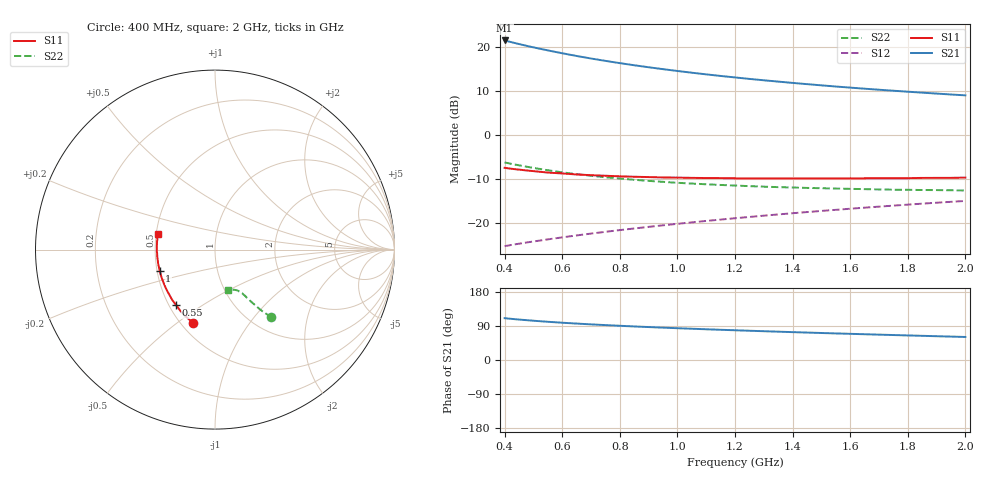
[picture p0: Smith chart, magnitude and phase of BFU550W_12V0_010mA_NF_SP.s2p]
! Filename:  P:\Prog\Test\Noise\ATS_data\Testdata_Net\06 Compressed Noise after Statistics\BFU550W_APM2013_11_D05_12p0V_010mA_NF_CM01_D.sf
! Date/Time: Tue 26/Mar/2013 16:25:26
! BFU550W_APM2013_11_D05_12p0V_1to35mA_NF_CM01_Bias6_R.sf
! Noise Parameter Data File
! BFU550W_APM2013_11_D05_12p0V_1to35mA_NF_CM01
! Date/time: Mon Mar 25 15:58:35 2013
! VAR V_out= 12.001000
! VAR I_out= 9.990000
! VAR V_in= 0.792300
! VAR I_in= 0.086905
! Device data file deembeded for feedlines and parallel
! Original file: \06 Compressed Noise after Statistics\BFU550W_APM2013_11_D05_12p0V_010mA_NF_CM01_R.sf
! Feed-files: PR019V01_070313_Feed1.s2p, PR019V01_070313_Feed2.s2p
! Parallel-file: PR019V01_070313_Par.s2p
# MHz S MA R 50
!  Freq-MHz  S11-mag  S11-arg  S21-mag  S21-arg  S12-mag  S12-arg  S22-mag  S22-arg
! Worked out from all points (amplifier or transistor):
!   37 points, 400 MHz to 2 GHz, reference 50 ohm
!   highest |S21| = 21.5 dB at 400 MHz (marker M1)
!   |S21| within 3 dB of that: start of sweep to 608.1 MHz
!   unconditionally stable (mu >= 1): 1.474 GHz to end of sweep
!   at 500 MHz: K = 0.72, MSG = 22.0 dB, |S12| = -24.1 dB
!   at 1.1 GHz: K = 0.96, MSG = 16.6 dB, |S12| = -19.4 dB
!   at 2 GHz: K = 1.01, MAG = 11.3 dB, |S12| = -14.9 dB
!   lowest NFmin = 0.73 dB at 420 MHz
!   S11 on the Smith chart (normalised r, x): 400 MHz: 0.57, -0.57; 550 MHz: 0.54, -0.39; 1 GHz: 0.52, -0.14; 2 GHz: 0.51, +0.10
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400  0.4265 -106.5  11.85 110.3  0.05524 58.0  0.4904 -50.1
420  0.4181 -109.3  11.4 108.8  0.05674 57.9  0.476 -50.7
440  0.4105 -112.1  10.99 107.4  0.0582 57.9  0.462 -51.3
460  0.4038 -114.7  10.6 106.1  0.05964 58.0  0.4491 -51.8
500  0.3914 -119.7  9.892 103.7  0.06244 58.2  0.4258 -52.7
550  0.377 -125.1  9.144 100.9  0.06595 58.6  0.4006 -53.6
600  0.3684 -130.2  8.482 98.4  0.06951 59.0  0.3792 -54.2
650  0.3589 -134.7  7.902 96.1  0.07309 59.4  0.3623 -54.9
700  0.3522 -139.0  7.397 94.0  0.07669 59.9  0.3469 -55.5
750  0.347 -142.8  6.952 92.1  0.08034 60.3  0.3337 -55.9
800  0.3417 -146.5  6.556 90.3  0.08401 60.7  0.3227 -56.5
850  0.338 -150.0  6.202 88.5  0.08766 61.1  0.3122 -56.8
950  0.3319 -155.9  5.601 85.4  0.09519 61.8  0.2959 -57.6
1000  0.3305 -158.7  5.343 83.9  0.09898 62.0  0.2887 -57.9
1100  0.3268 -163.8  4.891 81.1  0.1067 62.5  0.2778 -59.0
1200  0.3248 -168.4  4.513 78.5  0.1145 62.8  0.2687 -60.1
1250  0.3241 -170.8  4.343 77.2  0.1184 62.9  0.2645 -60.5
1350  0.3235 -174.6  4.047 74.7  0.1265 63.1  0.2578 -61.7
1500  0.3236 179.8  3.672 71.2  0.1386 63.0  0.2507 -63.7
1650  0.3248 174.6  3.364 68.0  0.1509 62.9  0.2447 -65.7
1750  0.3259 171.8  3.191 65.9  0.1591 62.7  0.2413 -67.2
2000  0.3306 164.5  2.828 60.8  0.1799 61.9  0.2365 -71.7
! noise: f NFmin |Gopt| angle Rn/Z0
400  0.7666  0.05367  148.1  0.0912
460  0.7746  0.08436  155.2  0.0817
600  0.7923  0.09056  154.6  0.0884
800  0.8317  0.1235  156.5  0.0789
1000  0.8535  0.1526  160.6  0.0757
1200  0.8716  0.1904  163.7  0.072
1400  0.9048  0.2117  170.2  0.072
1600  0.9391  0.2298  175  0.0697
1800  0.9835  0.2542  -177.6  0.0681
2000  1.024  0.2645  -174.4  0.0717
